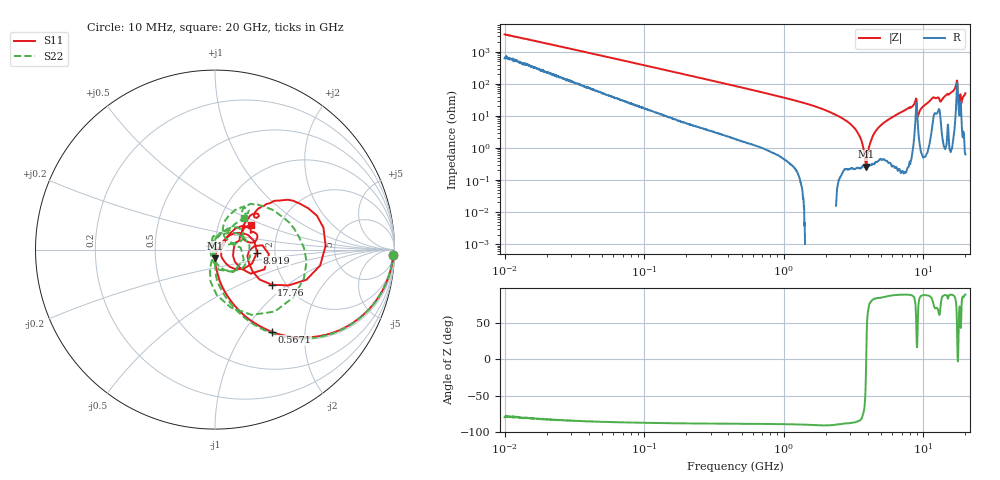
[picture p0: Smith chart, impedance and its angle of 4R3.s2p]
!Keysight Technologies,P5008B,MY61100088,A.16.20.02
!Date: Monday, October 30, 2023 16:42:54
!Correction: S11(C  2-Port  )
!S21(C  2-Port  )
!S12(C  2-Port  )
!S22(C  2-Port  )
!S2P File: Measurements: S11, S21, S12, S22:Log Frequency Sweep
# Hz S  dB  R 50
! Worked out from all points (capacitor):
!   1601 points, 10 MHz to 20 GHz, reference 50 ohm
!   read as one part in series: C = 4.57 pF near 10.39 MHz
!   lowest |Z| = 261 mohm at 3.902 GHz (marker M1)
!   series resonance near 3.893 GHz, so ESL is about 370 pH
!   S11 on the Smith chart (normalised r, x): 10 MHz: 12, -68; 567.1 MHz: 1.02, -1.36; 8.919 GHz: 1.61, -0.06; 17.76 GHz: 1.70, -0.77; 20 GHz: 1.43, +0.42
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1e7  -0.04 -1.6  -30.83 78.0  -30.83 78.1  -0.05 -1.6
3.555162e7  -0.11 -5.4  -20.44 79.7  -20.45 79.7  -0.11 -5.5
1.263918e8  -0.56 -18.2  -10.14 69.4  -10.15 69.4  -0.56 -18.4
4.472136e8  -3.79 -48.7  -2.52 39.7  -2.52 39.7  -3.79 -49.4
5.671164e8  -5.06 -55.2  -1.74 33.2  -1.75 33.2  -5.07 -56.2
1.589917e9  -12.92 -78.1  -0.22 11.0  -0.23 11.0  -12.90 -81.1
3.902191e9  -26.27 -88.9  -0.04 -2.9  -0.04 -2.9  -26.13 -92.0
4.948411e9  -33.97 -67.3  -0.02 -6.7  -0.03 -6.8  -35.30 -87.8
5.652411e9  -37.41 -15.0  -0.01 -9.1  -0.01 -9.1  -50.33 -165.2
6.611766e9  -30.04 30.4  -0.01 -12.2  -0.01 -12.2  -31.53 115.3
7.697294e9  -23.10 39.6  -0.03 -16.2  -0.03 -16.2  -23.63 102.9
8.344716e9  -23.02 45.5  -0.07 -19.2  -0.07 -19.3  -23.61 82.0
8.918577e9  -12.61 -4.1  -2.04 -19.6  -2.04 -19.6  -14.00 -12.2
9.39702e9  -27.31 -37.0  -0.09 -17.1  -0.10 -17.1  -34.83 -129.4
9.66872e9  -29.03 1.8  -0.03 -19.1  -0.04 -19.2  -35.68 119.7
1.163675e10  -13.79 40.4  -0.60 -30.2  -0.60 -30.3  -15.12 44.6
1.335558e10  -15.47 21.8  -0.55 -25.1  -0.55 -25.1  -19.68 64.9
1.592205e10  -9.09 42.8  -0.64 -42.9  -0.64 -42.9  -9.43 48.7
1.693636e10  -6.17 34.5  -1.86 -54.8  -1.87 -54.8  -7.11 19.9
1.776035e10  -8.62 -31.8  -2.76 -19.4  -2.76 -19.4  -11.96 -87.9
1.862442e10  -12.42 -34.0  -1.70 -28.7  -1.71 -28.7  -18.89 -80.0
2e10  -12.25 34.9  -0.35 -47.7  -0.35 -47.8  -12.42 47.6
